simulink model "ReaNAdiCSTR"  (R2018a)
settings: Solver=VariableStepAuto  StartTime=0.0  StopTime=10  RelTol=1e-3
undefined symbols (not defined in the file): a4aaa25c, ab00, b3eaa3b65f8c, c2d0, d692ba2f46fd, e43d8a497eb3, e93df6e6, ea73, ReaNAdiCSTR, sdiscope

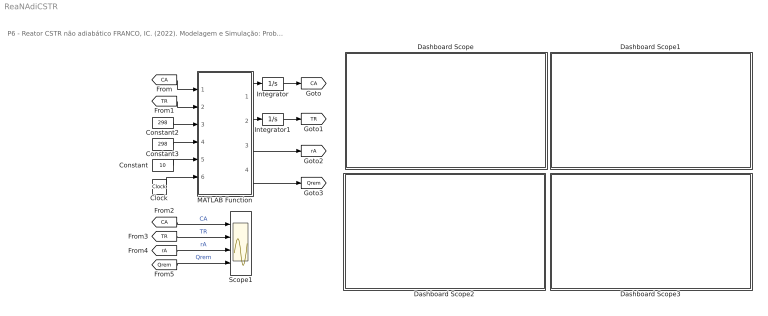
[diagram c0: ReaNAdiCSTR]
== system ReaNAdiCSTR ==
  note: P6 - Reator CSTR não adiabático FRANCO, IC. (2022). Modelagem e Simulação: Problemas Típicos da Engenharia Química para Simulação e Análise. NOTAS DE AULA INOVADORAS. The Journal of Engineering and Exact Sciences. Material Complementar.
  Clock : Clock
  Constant : Constant  Value=10
  Constant2 : Constant  Value=298
  Constant3 : Constant  Value=298
  Dashboard Scope : Subsystem  DialogController=hmiCreateDDGDialog  IsWebBlock=on  mask(MWDashboardBlock){webBlockId=38deba12-ea73-4d11-ab00-34912660ab8e, webBlockType=sdiscope, ShowInitialText=on, HMISrcModelName=ReaNAdiCSTR}
      mask prompts: webBlockId "WebBlock Id"; webBlockType "WebBlock Type"; HMISrcModelName "Source Model"
      mask help: SimulinkHMI:dialogs:HMIScopeDialogDesc
  Dashboard Scope1 : Subsystem  DialogController=hmiCreateDDGDialog  IsWebBlock=on  mask(MWDashboardBlock){webBlockId=985579e3-e327-476c-9c10-b3eaa3b65f8c, webBlockType=sdiscope, ShowInitialText=on, HMISrcModelName=ReaNAdiCSTR}
      mask prompts: webBlockId "WebBlock Id"; webBlockType "WebBlock Type"; HMISrcModelName "Source Model"
      mask help: SimulinkHMI:dialogs:HMIScopeDialogDesc
  Dashboard Scope2 : Subsystem  DialogController=hmiCreateDDGDialog  IsWebBlock=on  mask(MWDashboardBlock){webBlockId=e93df6e6-c2d0-42d7-8e0a-e43d8a497eb3, webBlockType=sdiscope, ShowInitialText=on, HMISrcModelName=ReaNAdiCSTR}
      mask prompts: webBlockId "WebBlock Id"; webBlockType "WebBlock Type"; HMISrcModelName "Source Model"
      mask help: SimulinkHMI:dialogs:HMIScopeDialogDesc
  Dashboard Scope3 : Subsystem  DialogController=hmiCreateDDGDialog  IsWebBlock=on  mask(MWDashboardBlock){webBlockId=a4aaa25c-0956-4708-8470-d692ba2f46fd, webBlockType=sdiscope, ShowInitialText=on, HMISrcModelName=ReaNAdiCSTR}
      mask prompts: webBlockId "WebBlock Id"; webBlockType "WebBlock Type"; HMISrcModelName "Source Model"
      mask help: SimulinkHMI:dialogs:HMIScopeDialogDesc
  Integrator : Integrator  InitialCondition=10
  Integrator1 : Integrator  InitialCondition=298
  MATLAB Function : MATLAB Function  TreatAsAtomicUnit=on
  Scope1 : Scope  NumInputPorts=4
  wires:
  MATLAB Function/4(Qrem) -> [Qrem]
  MATLAB Function/3(rA) -> [rA]
  Constant3/1 -> MATLAB Function/4(Tj)
  Clock/1 -> MATLAB Function/6(t)
  Constant/1 -> MATLAB Function/5(CA0)
  Constant2/1 -> MATLAB Function/3(T0)
  MATLAB Function/2(dTR) -> Integrator1/1
  [CA] -> MATLAB Function/1(CA)
  Integrator/1 -> [CA]
  Integrator1/1 -> [TR]
  [TR] -> MATLAB Function/2(TR)
  MATLAB Function/1(dCA) -> Integrator/1
  [CA] -> Scope1/1  "CA"
  [TR] -> Scope1/2  "TR"
  [rA] -> Scope1/3  "rA"
  [Qrem] -> Scope1/4  "Qrem"

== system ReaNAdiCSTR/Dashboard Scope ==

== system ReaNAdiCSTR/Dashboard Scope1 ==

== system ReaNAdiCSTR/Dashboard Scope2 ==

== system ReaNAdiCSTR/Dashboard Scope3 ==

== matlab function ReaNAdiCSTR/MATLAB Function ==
function [dCA,dTR,rA,Qrem] = fcn(CA,TR,T0,Tj,CA0,t)
%% Parâmetros
Ea  = 11843.000;
k0  = 14825.000*3600;
R   =     1.987;
UApV=   250.000;
dH  =  5215.000;
rCp =   500.000;
tau =     1.000;

%% equações auxiliares
k   = k0*exp(-Ea/(R*TR));
rA  = k*CA;
Qrem= UApV*(TR-Tj);

%% Modelo matemático
dCA = (1/tau)*CA0-(1/tau)*CA-rA;
dTR = (1/tau)*(T0-TR)-rA*(-dH)/rCp-Qrem/rCp;
end
